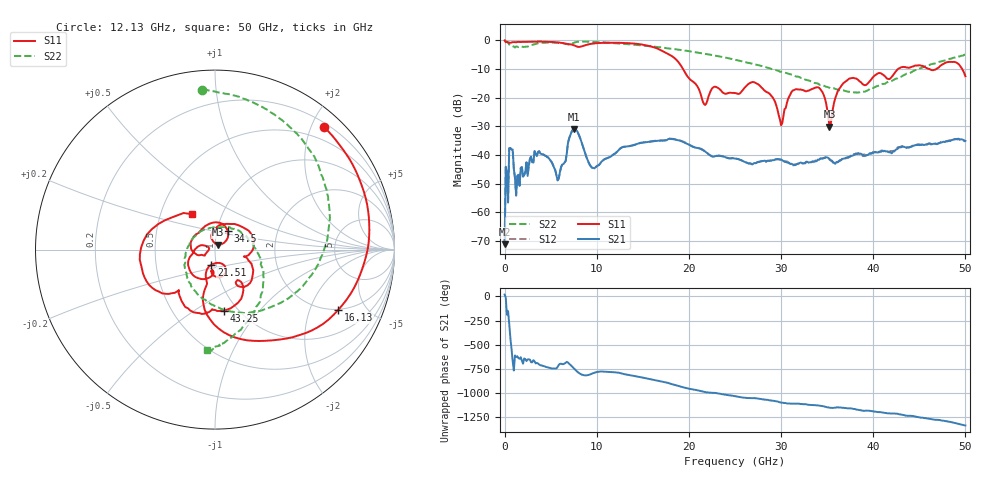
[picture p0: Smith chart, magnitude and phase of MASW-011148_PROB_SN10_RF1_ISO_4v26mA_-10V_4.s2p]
!Keysight Technologies,N5247A,US51170177,A.10.64.09
!Date: Saturday, May 29, 2021 13:32:36
!Correction: S11(Full 2 Port(1,2))
!S21(Full 2 Port(1,2))
!S12(Full 2 Port(1,2))
!S22(Full 2 Port(1,2))
!S2P File: Measurements: S11, S21, S12, S22:
# Hz S  dB  R 50
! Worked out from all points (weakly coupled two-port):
!   401 points, 10 MHz to 50 GHz, reference 50 ohm
!   highest |S21| = -31.04 dB at 7.508 GHz (marker M1); lowest = -71.2 dB at 10 MHz (marker M2)
!   lowest |S11| = -30.1 dB at 35.25 GHz (marker M3), VSWR 1.06, Z = 51.6 + j2.74 ohm
!   |S11| at or under -10 dB: 19.37 GHz to 42.68 GHz (23.32 GHz wide, 75.1 % of centre); 46.1 GHz to 46.82 GHz (720.5 MHz wide, 1.55 % of centre); 49.65 GHz to end of sweep
!   |S22| runs from -18.2 to 0.0 dB; largest |S21 - S12| = 0.0013
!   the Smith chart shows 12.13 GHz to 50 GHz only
!   S11 on the Smith chart (normalised r, x): 12.13 GHz: 0.27, +2.20; 16.13 GHz: 1.97, -3.19; 21.51 GHz: 0.95, -0.16; 34.5 GHz: 1.13, +0.23; 43.25 GHz: 0.86, -0.67; 50 GHz: 0.72, +0.30
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1e7  -0.01 -1.8  -71.23 18.4  -71.82 88.0  -0.02 -1.0
7.5985e8  -0.74 -87.4  -38.06 177.4  -38.05 177.8  -1.87 -55.4
1.384725e9  -0.53 -127.5  -47.33 100.5  -47.34 100.2  -2.14 -84.5
2.384525e9  -0.50 -163.9  -42.55 51.3  -42.58 50.9  -2.18 -117.5
5.883825e9  -0.72 128.9  -48.22 11.9  -48.18 11.2  -0.86 170.0
7.5085e9  -1.67 106.0  -31.04 -23.4  -31.02 -23.4  -0.84 153.9
8.383325e9  -2.06 102.5  -35.75 -88.9  -35.76 -88.9  -0.40 140.0
9.633075e9  -1.08 87.1  -44.49 -73.4  -44.47 -73.0  -0.49 123.4
1.213258e10  -0.78 48.3  -39.08 -66.0  -39.07 -66.1  -0.99 94.5
1.613178e10  -2.33 -26.0  -35.20 -141.9  -35.12 -141.3  -2.12 52.1
1.675665e10  -3.09 -40.2  -34.99 -155.2  -34.90 -154.7  -2.34 45.7
2.15057e10  -21.28 -103.9  -38.26 96.5  -38.16 96.2  -4.53 -3.9
2.5005e10  -18.39 -99.8  -41.25 48.9  -41.16 48.7  -6.74 -41.9
2.737952e10  -15.10 -146.3  -42.54 25.8  -42.62 24.0  -8.53 -69.3
3.0004e10  -29.62 167.3  -41.58 -16.9  -41.60 -16.5  -10.93 -102.1
3.337832e10  -16.92 111.9  -42.31 -42.8  -42.31 -43.1  -14.37 -153.4
3.45031e10  -18.13 55.0  -41.12 -54.3  -41.31 -55.1  -15.62 -172.2
3.525295e10  -30.14 58.6  -41.36 -70.7  -41.55 -68.7  -16.50 172.0
3.725255e10  -13.68 33.5  -40.70 -77.6  -41.08 -77.0  -17.89 125.8
4.175165e10  -13.52 -53.5  -39.06 -128.7  -38.80 -129.2  -14.32 19.1
4.325135e10  -9.24 -82.0  -37.15 -145.2  -36.94 -147.2  -12.24 -6.4
5e10  -12.52 123.4  -35.04 106.0  -35.27 105.4  -5.00 -94.7
